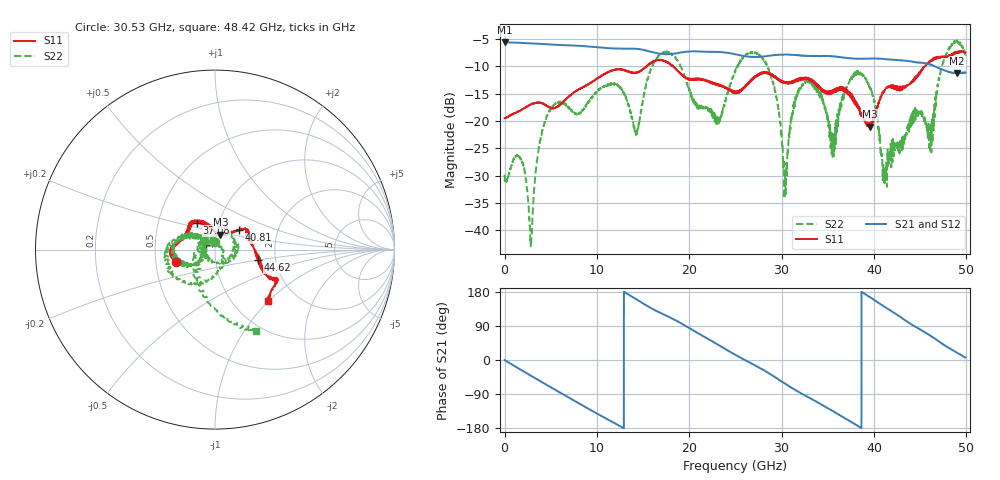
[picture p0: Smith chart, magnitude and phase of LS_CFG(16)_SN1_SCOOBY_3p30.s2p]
!Keysight Technologies,N5245B,MY58422026,A.13.80.08
!Date: Thursday, March 19, 2020 23:31:42
!Correction: S11(Full 2 Port(1,2))
!S21(Full 2 Port(1,2))
!S12(Full 2 Port(1,2))
!S22(Full 2 Port(1,2))
!S2P File: Measurements: S11, S21, S12, S22:
# Hz S DB R 50.0
!freq dBS11 angS11 dBS21 angS21 dBS12 angS12 dBS22 angS22
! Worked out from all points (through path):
!   4991 points, 10 MHz to 49.91 GHz, reference 50 ohm
!   highest |S21| = -5.54 dB at 10 MHz (marker M1); lowest = -11.2 dB at 49.02 GHz (marker M2)
!   group delay of S21, straight-line fit = 39.3 ps
!   lowest |S11| = -21.0 dB at 39.61 GHz (marker M3), VSWR 1.20, Z = 52.3 + j8.85 ohm
!   |S11| at or under -10 dB: start of sweep to 15.34 GHz; 18.27 GHz to 45.5 GHz (27.23 GHz wide, 85.4 % of centre)
!   |S22| runs from -42.9 to -5.2 dB; largest |S21 - S12| = 0.005
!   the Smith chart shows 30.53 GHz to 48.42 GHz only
!   S11 on the Smith chart (normalised r, x): 30.53 GHz: 0.64, -0.09; 37.08 GHz: 0.79, +0.24; 40.81 GHz: 1.27, +0.28; 44.62 GHz: 1.62, -0.20; 48.42 GHz: 1.42, -0.99
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1e7  -19.47 -2.1  -5.54 -0.3  -5.53 -0.3  -29.82 2.1
1.77e9  -18.00 -21.8  -5.67 -25.8  -5.66 -25.8  -26.93 -32.2
2.86e9  -16.92 -32.0  -5.76 -41.4  -5.76 -41.4  -42.28 -81.6
4.64e9  -17.25 -51.1  -5.93 -66.8  -5.92 -66.7  -18.89 -122.1
8.33e9  -13.99 -68.5  -6.24 -118.3  -6.23 -118.3  -18.27 -86.0
1.427e10  -11.09 -114.8  -6.76 160.5  -6.76 160.5  -21.94 -127.9
1.665e10  -8.82 -126.5  -7.61 127.0  -7.60 127.0  -8.13 -163.6
2.301e10  -13.40 -148.5  -7.33 42.0  -7.32 42.1  -20.50 -165.7
2.496e10  -14.77 -141.8  -7.73 14.2  -7.72 14.3  -11.04 -172.6
2.831e10  -11.22 -155.8  -8.10 -30.4  -8.11 -30.2  -9.53 -83.6
3.053e10  -12.88 -162.8  -7.81 -64.8  -7.81 -64.6  -27.82 93.5
3.328e10  -12.48 175.1  -8.07 -103.6  -8.07 -103.2  -12.70 -166.9
3.554e10  -14.57 140.4  -8.11 -134.7  -8.05 -134.3  -26.55 -179.6
3.708e10  -14.94 123.7  -8.44 -156.8  -8.36 -156.8  -13.78 158.5
3.961e10  -21.01 70.5  -8.53 165.1  -8.52 164.9  -14.09 -112.7
4.081e10  -15.34 38.9  -8.58 146.0  -8.59 145.7  -26.32 -31.7
4.16e10  -13.60 33.9  -8.70 133.6  -8.72 133.4  -25.61 117.7
4.462e10  -12.08 -13.5  -9.27 85.9  -9.29 85.9  -18.43 20.0
4.615e10  -8.95 -27.3  -9.66 63.5  -9.68 63.5  -20.97 146.3
4.842e10  -7.71 -44.6  -11.14 27.7  -11.17 27.6  -5.87 -63.2
4.902e10  -7.26 -50.3  -11.21 18.9  -11.23 18.9  -5.28 -41.9
4.991e10  -7.50 -49.7  -11.11 6.7  -11.13 6.6  -7.80 -16.0
